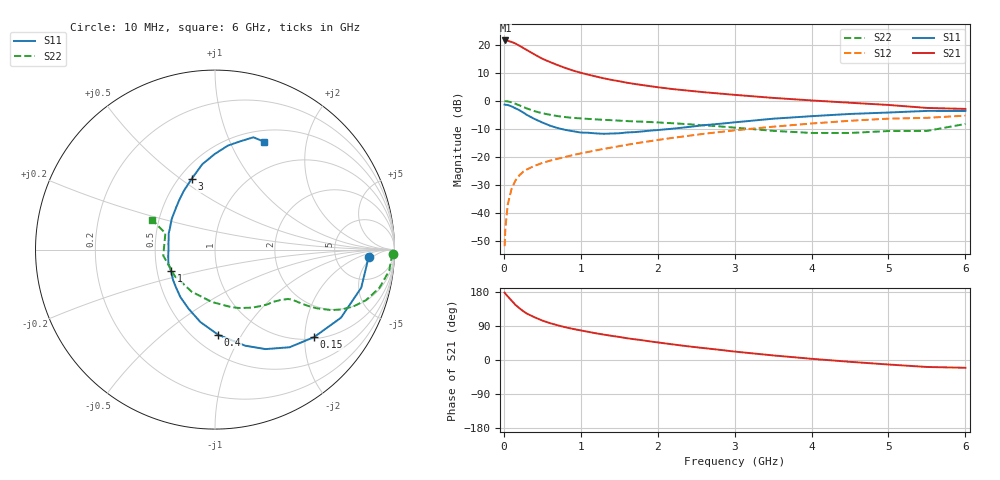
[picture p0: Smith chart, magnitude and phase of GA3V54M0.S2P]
! Infineon Technologies  Discrete & RF Semiconductors
! BF775
! Si NPN RF Bipolar Junction Transistor in SOT23
! VCE = 3.5 V  IC = 4 mA
! Common Emitter S-Parameters:  May  1996
# GHz  S  MA  R  50
!  f  S11  S21  S12  S22
! GHz  MAG  ANG  MAG  ANG  MAG  ANG  MAG  ANG
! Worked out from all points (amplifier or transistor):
!   36 points, 10 MHz to 6 GHz, reference 50 ohm
!   highest |S21| = 21.5 dB at 20 MHz (marker M1)
!   |S21| within 3 dB of that: start of sweep to 273.4 MHz
!   unconditionally stable (mu >= 1): 877.8 MHz to 3.493 GHz
!   at 250 MHz: K = 0.42, MSG = 22.0 dB, |S12| = -25.3 dB
!   at 1.4 GHz: K = 1.12, MAG = 9.9 dB, |S12| = -16.6 dB
!   at 6 GHz: K = 0.96, MSG = 1.2 dB, |S12| = -5.3 dB
!   S11 on the Smith chart (normalised r, x): 10 MHz: 12, -4; 150 MHz: 1.05, -2.23; 400 MHz: 0.65, -0.80; 1 GHz: 0.59, -0.15; 3 GHz: 0.58, +0.55; 6 GHz: 0.63, +1.35
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0.01  0.8566 -2.9  11.78 177.7  0.0026 89.7  0.9936 -1.4
0.02  0.8495 -5.9  11.84 174.9  0.0053 84.5  0.9843 -2.8
0.05  0.842 -14.6  11.68 168.0  0.0141 82.9  0.9777 -6.9
0.1  0.7979 -28.4  11.15 156.9  0.0271 75.4  0.9407 -13.1
0.15  0.7367 -41.4  10.45 145.6  0.038 68.7  0.8875 -18.5
0.2  0.6848 -52.6  9.581 137.1  0.047 64.0  0.8325 -22.4
0.25  0.6216 -63.1  8.747 129.1  0.0546 60.3  0.7802 -25.3
0.3  0.561 -72.6  7.99 122.4  0.0602 58.2  0.7301 -27.5
0.4  0.4746 -87.9  6.66 112.7  0.0699 54.9  0.6536 -30.0
0.5  0.4118 -101.4  5.607 104.1  0.0785 53.7  0.6011 -31.3
0.6  0.3611 -114.0  4.895 97.3  0.0862 53.0  0.5644 -32.0
0.7  0.3279 -125.9  4.314 91.5  0.0931 53.5  0.535 -32.5
0.8  0.3039 -135.3  3.838 86.4  0.1008 53.6  0.5133 -33.0
1  0.2726 -154.2  3.152 78.0  0.1161 54.2  0.4866 -34.5
1.1  0.2705 -163.5  2.911 74.2  0.1236 54.5  0.4765 -35.7
1.6  0.2736 160.4  2.097 57.4  0.1652 54.6  0.4362 -41.8
2.2  0.3197 132.6  1.614 41.1  0.22 52.0  0.3986 -52.7
3  0.4143 108.4  1.277 22.2  0.2984 45.2  0.3338 -74.0
3.5  0.4806 98.5  1.127 12.1  0.3464 39.6  0.2923 -93.4
4.5  0.5841 82.9  0.924 -4.8  0.4417 26.9  0.2682 -147.0
5.5  0.6615 71.1  0.747 -18.4  0.498 11.7  0.2913 161.7
6  0.6602 65.6  0.718 -20.5  0.5449 7.5  0.3877 154.6
